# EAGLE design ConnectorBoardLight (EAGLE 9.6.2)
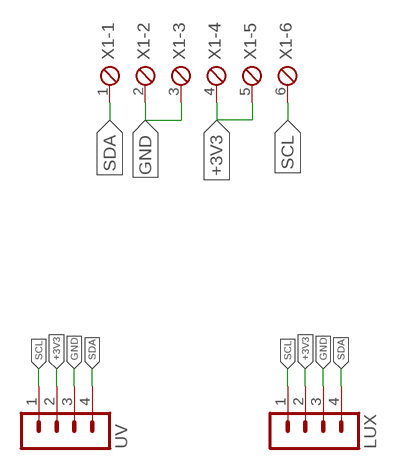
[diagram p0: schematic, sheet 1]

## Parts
LUX  B4B-PH-K-S  [B4B-PH-K-S]
UV  B4B-PH-K-S  [B4B-PH-K-S]
X1  MPT6  [6POL254]

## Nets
+3V3: LUX.2 UV.2 X1.4 X1.5
GND: LUX.3 UV.3 X1.2 X1.3
SCL: LUX.1 UV.1 X1.6
SDA: LUX.4 UV.4 X1.1

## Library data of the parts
LUX UV = con-JSTPH:B4B-PH: JST PH series header 2.00mm pitch disconnectable crimp style connectors, vertical (side entry type), 4 pins
X1 = con-phoenix-254:MPT6: PHOENIX CONNECTOR; OC_FARNELL: unknown; OC_NEWARK: unknown

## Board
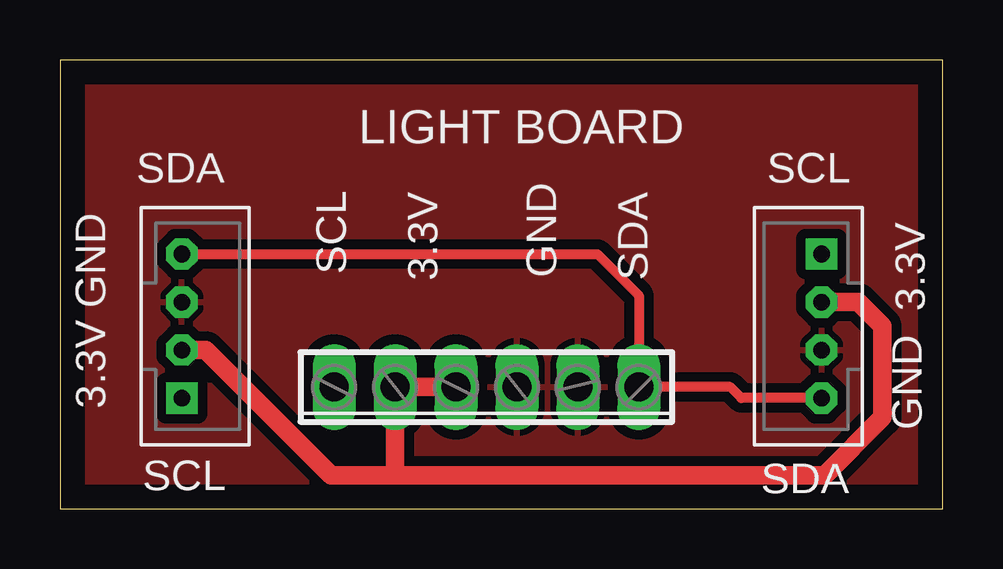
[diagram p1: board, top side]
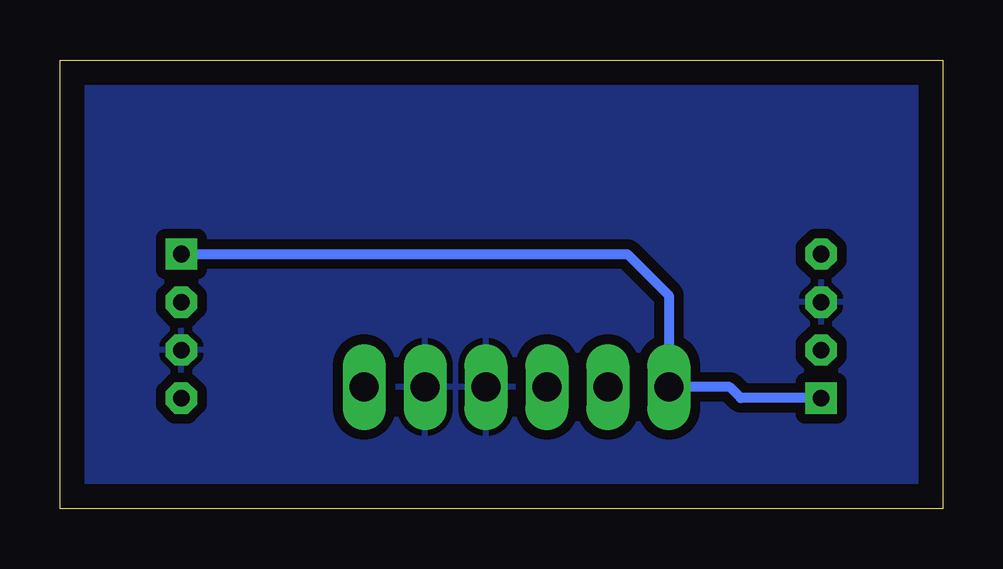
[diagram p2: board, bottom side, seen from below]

Size 36.81 x 18.72 mm. Coordinates in mm from the lower left corner, seen from the top.
Outline: 0,0 36.81,0 36.81,18.72 0,18.72 0,0
Copper layers (1*16): Top 0.035mm / dielectric 1.5mm / Bottom 0.035mm
Design rules "default": minimum track width 6mil, minimum drill 0.35mm, track to track 6mil, track to pad 6mil, pad to pad 6mil, via to via 6mil, smd to smd 6mil, copper to edge 40mil, drill to drill 6mil, minimum pad ring 10mil, minimum via ring 8mil, stop-mask expansion 4mil, vias tented up to drill 0mil, thermal gap 10mil

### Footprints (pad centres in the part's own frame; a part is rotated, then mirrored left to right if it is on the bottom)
B4B-PH-K-S = drill 0.7 pad 1.3 square: 1 3,0 | drill 0.7 pad 1.3 octagon: 2 1,0; 3 -1,0; 4 -3,0
6POL254 = drill 1.2 pad 1.778 long: 1 -6.35,0; 2 -3.81,0; 3 -1.27,0; 4 1.27,0; 5 3.81,0; 6 6.35,0

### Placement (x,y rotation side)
LUX  5.08,7.62 270 top
UV  31.75,7.62 90 top
X1  17.78,5.08 180 top

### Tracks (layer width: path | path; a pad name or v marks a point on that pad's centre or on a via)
+3V3
  Top 0.762: LUX.2 6.08,6.62 11.3,1.4 13.97,1.4 | X1.4 X1.5 13.97,1.4 | UV.2 33.29,8.62 34.29,7.62 34.29,3.81 31.88,1.4 13.97,1.4
GND
  pour Top (isolate 0.406): 0,19.05 36.83,19.05 36.83,0 0,0
  pour Bottom (isolate 0.406): 0,19.05 36.83,19.05 36.83,0 0,0
SCL
  Bottom 0.406: LUX.1 8.43,4.62 8.89,5.08 X1.6 11.43,8.89 13.16,10.62 UV.1
SDA
  Top 0.406: UV.4 28.4,4.62 27.94,5.08 X1.1 24.13,8.89 22.4,10.62 LUX.4

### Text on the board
tPlace: SDA | LIGHT BOARD | SCL | SDA | SCL | 3.3V | GND | GND | 3.3V | 3.3V | GND | SCL | SDA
